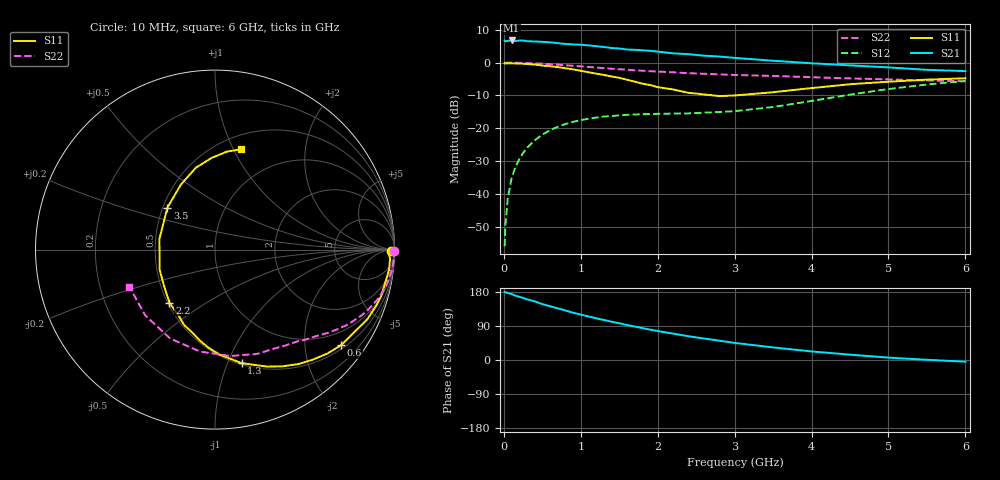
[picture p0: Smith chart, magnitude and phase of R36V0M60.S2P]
! SIEMENS Small Signal Semiconductors
! BFR181
! Si NPN RF Bipolar Junction Transistor in SOT23
! VCE = 6 V  IC = 0.6 mA
! Common Emitter S-Parameters:  May  1996
# GHz  S  MA  R  50
!  f  S11  S21  S12  S22
! GHz  MAG  ANG  MAG  ANG  MAG  ANG  MAG  ANG
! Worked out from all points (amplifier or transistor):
!   36 points, 10 MHz to 6 GHz, reference 50 ohm
!   highest |S21| = 6.7 dB at 100 MHz (marker M1)
!   |S21| within 3 dB of that: start of sweep to 1.803 GHz
!   unconditionally stable (mu >= 1): 2.306 GHz to 3.894 GHz
!   at 250 MHz: K = 0.12, MSG = 17.1 dB, |S12| = -27.6 dB
!   at 1.4 GHz: K = 0.64, MSG = 10.4 dB, |S12| = -16.3 dB
!   at 6 GHz: K = 0.90, MSG = 1.5 dB, |S12| = -5.6 dB
!   S11 on the Smith chart (normalised r, x): 10 MHz: 74, -35; 600 MHz: 0.60, -2.87; 1.3 GHz: 0.51, -1.12; 2.2 GHz: 0.51, -0.36; 3.5 GHz: 0.53, +0.28; 6 GHz: 0.64, +1.07
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0.01  0.978 -0.6  2.17 179.6  0.0016 94.9  0.9996 -0.4
0.02  0.9694 -1.4  2.108 178.6  0.0033 86.5  0.9909 -0.7
0.05  0.9768 -3.0  2.147 176.9  0.0084 87.4  0.9984 -1.5
0.1  0.9763 -6.4  2.174 174.1  0.0171 85.3  0.9999 -2.9
0.15  0.9699 -9.1  2.126 169.9  0.0256 83.2  0.9945 -4.6
0.2  0.9642 -12.5  2.166 166.8  0.0337 81.4  0.9919 -5.9
0.25  0.9612 -15.7  2.173 163.8  0.0419 79.0  0.9892 -7.5
0.3  0.9523 -18.9  2.122 160.2  0.0501 77.3  0.9836 -8.9
0.5  0.9008 -30.9  2.072 147.5  0.0797 69.1  0.9609 -14.5
0.6  0.8819 -37.1  2.038 141.9  0.0933 65.0  0.9458 -17.2
0.9  0.7892 -53.9  1.895 124.8  0.1253 54.9  0.8957 -24.1
1.1  0.7141 -65.9  1.831 115.0  0.14 49.5  0.8585 -28.3
1.3  0.6495 -76.8  1.729 105.6  0.1506 44.9  0.8235 -31.9
1.6  0.5485 -93.7  1.581 92.3  0.1603 40.1  0.7805 -36.5
1.8  0.4773 -105.7  1.54 84.3  0.1642 38.5  0.7528 -39.3
2.2  0.3897 -130.7  1.383 69.6  0.1673 37.1  0.7112 -44.9
2.4  0.3466 -145.6  1.344 62.7  0.1683 38.4  0.6895 -47.7
2.8  0.309 -176.7  1.237 51.0  0.1768 41.5  0.6626 -53.8
3.5  0.3539 138.5  1.067 33.2  0.2106 48.8  0.627 -67.9
4.5  0.4686 103.1  0.907 14.1  0.3255 49.6  0.5744 -98.1
5.5  0.5502 83.0  0.776 0.6  0.464 37.3  0.5342 -136.6
6  0.5773 75.4  0.742 -4.5  0.5252 28.9  0.5199 -156.6
